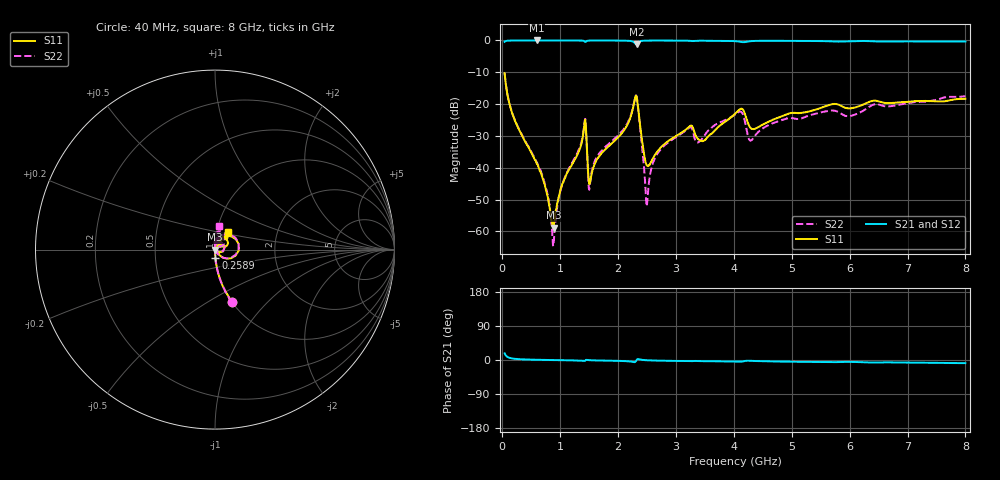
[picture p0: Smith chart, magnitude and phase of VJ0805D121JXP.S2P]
! VJ0805D121JXP
! DATE 03/14/2022  08:52
! CAPACITORS MOUNTED IN SERIES ON 25 MIL THICK MICROSTRIP SUBSTRATE
# GHz  S  MA  R  50.00
!  FREQ  S11M  S11A  S21M  S21A  S12M  S12A  S22M  S22A
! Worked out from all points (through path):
!   801 points, 40 MHz to 8 GHz, reference 50 ohm
!   highest |S21| = 0.00 dB at 597.2 MHz (marker M1); lowest = -1.2 dB at 2.319 GHz (marker M2)
!   group delay of S21, straight-line fit = 3.38 ps
!   lowest |S11| = -58.8 dB at 885.8 MHz (marker M3), VSWR 1.00, Z = 50.1 + j0.0241 ohm
!   |S11| at or under -10 dB: start of sweep to end of sweep
!   |S22| runs from -64.7 to -10.2 dB; largest |S21 - S12| = 0.0041
!   S11 on the Smith chart (normalised r, x): 40 MHz: 1.00, -0.64; 258.9 MHz: 1.00, -0.09; 8 GHz: 1.13, +0.22
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0.04  0.3047 -72.1  0.9515 17.7  0.9499 17.7  0.3073 -72.5
0.2589  0.04505 -87.3  0.9987 2.6  0.9989 2.5  0.04573 -87.6
0.5972  0.0115 -85.5  0.9995 0.6  0.9997 0.6  0.01206 -87.7
0.7564  0.004366 -79.4  0.9992 0.1  1 0.1  0.004659 -83.8
0.88575  0.001146 12.1  0.9986 -0.2  0.9998 -0.2  0.0005855 3.1
1.02505  0.005056 71.1  0.9986 -0.5  0.9998 -0.6  0.005117 80.3
1.3733  0.02525 73.7  0.9942 -1.8  0.9951 -1.8  0.0268 79.1
1.42305  0.05246 41.2  0.9619 -2.6  0.9631 -2.6  0.05454 45.2
1.52255  0.006346 45.7  0.9964 -0.7  0.9972 -0.7  0.006377 67.4
1.64195  0.01386 73.0  0.9976 -1.2  0.9987 -1.3  0.01521 85.3
2.09965  0.03828 73.2  0.9934 -2.8  0.9941 -2.8  0.04075 83.8
2.31855  0.1324 -2.5  0.868 -0.6  0.8693 -0.6  0.1323 0.9
2.49765  0.01089 -3.7  0.9937 -0.7  0.9951 -0.7  0.002472 23.9
2.69665  0.01895 54.9  0.9951 -1.7  0.9967 -1.7  0.01762 90.7
3.2439  0.04529 45.0  0.9849 -3.2  0.9868 -3.2  0.04312 72.6
3.4827  0.02657 54.1  0.9886 -3.1  0.9897 -3.2  0.03123 94.7
4.02995  0.0718 57.0  0.9734 -4.6  0.9745 -4.7  0.06954 73.3
4.1394  0.08434 34.5  0.9423 -4.1  0.944 -4.1  0.07355 46.8
4.2986  0.04142 28.6  0.976 -2.2  0.9773 -2.3  0.02679 62.5
5.3533  0.07863 54.1  0.9798 -5.0  0.9803 -5.1  0.0683 86.0
6.67665  0.1037 52.9  0.9649 -6.3  0.9663 -6.4  0.09196 75.4
8  0.1213 53.7  0.9607 -8.3  0.9617 -8.4  0.1327 79.2
